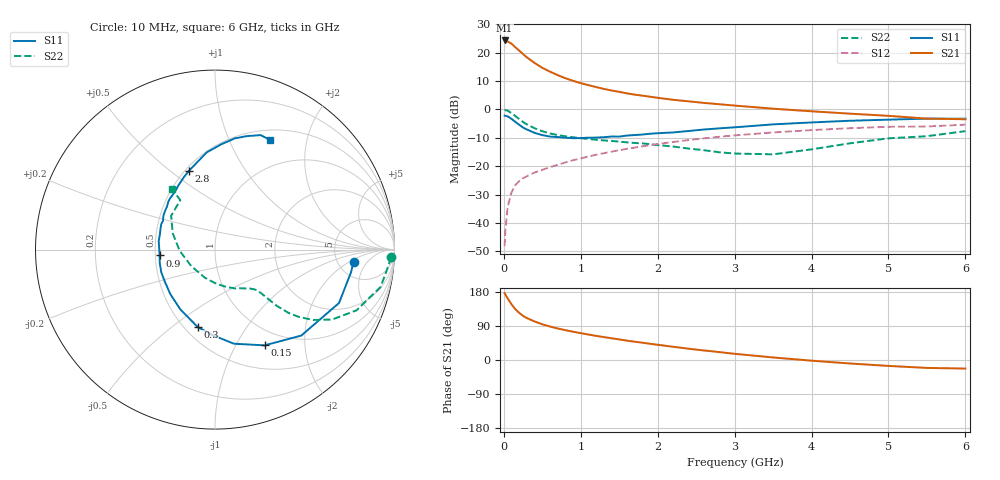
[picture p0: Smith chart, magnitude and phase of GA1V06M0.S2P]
! Infineon Technologies  Discrete & RF Semiconductors
! BF775
! Si NPN RF Bipolar Junction Transistor in SOT23
! VCE = 1 V  IC = 6 mA
! Common Emitter S-Parameters:  May  1996
# GHz  S  MA  R  50
!  f  S11  S21  S12  S22
! GHz  MAG  ANG  MAG  ANG  MAG  ANG  MAG  ANG
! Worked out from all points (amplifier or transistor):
!   36 points, 10 MHz to 6 GHz, reference 50 ohm
!   highest |S21| = 24.2 dB at 10 MHz (marker M1)
!   |S21| within 3 dB of that: start of sweep to 175.2 MHz
!   unconditionally stable (mu >= 1): 641.8 MHz to end of sweep
!   at 250 MHz: K = 0.57, MSG = 21.9 dB, |S12| = -24.3 dB
!   at 1.4 GHz: K = 1.17, MAG = 8.3 dB, |S12| = -14.9 dB
!   at 6 GHz: K = 1.03, MAG = -0.2 dB, |S12| = -5.4 dB
!   S11 on the Smith chart (normalised r, x): 10 MHz: 7.07, -2.39; 150 MHz: 0.79, -1.32; 300 MHz: 0.58, -0.62; 900 MHz: 0.53, -0.04; 2.8 GHz: 0.52, +0.58; 6 GHz: 0.62, +1.43
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0.01  0.775 -5.0  16.31 176.4  0.0039 87.7  0.9815 -2.5
0.02  0.768 -9.6  16.14 172.6  0.0075 84.6  0.9709 -5.2
0.05  0.7522 -23.3  15.68 162.4  0.0193 76.8  0.946 -12.7
0.1  0.6787 -44.9  14.27 146.9  0.0345 68.9  0.8583 -23.2
0.15  0.6009 -62.6  12.37 133.9  0.0465 61.3  0.7605 -30.8
0.2  0.5349 -78.6  10.78 124.3  0.0548 57.6  0.6733 -35.6
0.25  0.4777 -91.3  9.372 116.4  0.0611 54.6  0.5982 -38.8
0.3  0.4416 -102.7  8.204 110.5  0.0665 54.0  0.5416 -40.7
0.4  0.3848 -120.2  6.55 101.7  0.077 52.9  0.465 -42.3
0.5  0.3514 -135.1  5.378 94.2  0.0862 53.5  0.4116 -42.8
0.6  0.3317 -147.4  4.599 88.3  0.0957 54.0  0.3763 -43.1
0.7  0.3249 -157.2  4.003 83.2  0.1055 54.8  0.3527 -43.4
0.9  0.3104 -174.0  3.174 74.6  0.127 55.1  0.322 -44.5
1.1  0.3174 171.3  2.663 67.2  0.1477 55.2  0.3009 -46.8
1.3  0.3231 160.7  2.289 60.5  0.169 54.3  0.2834 -49.6
1.6  0.3453 146.2  1.908 51.1  0.2017 52.4  0.2622 -55.3
2.2  0.3917 124.9  1.472 34.9  0.2657 46.7  0.2215 -71.6
2.8  0.4623 108.3  1.23 20.9  0.3288 39.6  0.1755 -97.9
3.5  0.5434 94.9  1.026 6.7  0.3915 30.2  0.1613 -145.5
4.5  0.6296 79.9  0.839 -9.2  0.4654 16.7  0.2525 158.9
5.5  0.6865 68.3  0.686 -20.9  0.4988 2.8  0.3364 125.1
6  0.6837 63.5  0.669 -22.6  0.5367 -1.0  0.4131 125.3
